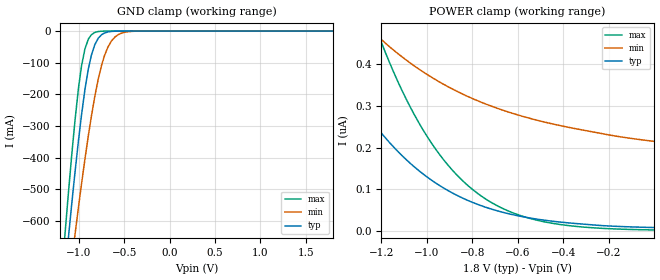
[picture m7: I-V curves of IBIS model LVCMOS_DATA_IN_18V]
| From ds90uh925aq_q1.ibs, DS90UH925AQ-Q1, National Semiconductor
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[Model] LVCMOS_DATA_IN_18V
Model_type Input
Vinh = 1.17V
Vinl = 0.63V
C_comp   6.98pF   6.05pF   8.06pF
[Voltage Range]   1.8V   1.62V   1.98V
[Temperature Range]   25.0   130.0   -40.0
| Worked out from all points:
|   GND clamp passes 1 mA (typ) near -0.64 V on its own axis
[GND Clamp]
-1.8V     -2.96A     -2.635A    -3.228A
-1.147V   -756.9mA   -899mA     -630.1mA
-1.114V   -658.8mA   -819.7mA   -517.7mA
-1.076V   -548.3mA   -728.9mA   -393.4mA
-1.039V   -442.8mA   -640.4mA   -278.7mA
-968.4mV  -265.6mA   -483.8mA   -110.5mA
-892.8mV  -119mA     -330.2mA   -25.29mA
-822.6mV  -43.26mA   -207.4mA   -4.329mA
-747mV    -11.35mA   -107.3mA   -370.4uA
-676.8mV  -2.58mA    -49.95mA   -28.17uA
-493.2mV  -19.24uA   -3.72mA    -1.533uA
1.796V    8.087nA    0A         1.419nA
[POWER Clamp]
-1.8V     917.5nA    912.1nA    12.77uA
-1.487V   487.3nA    635.3nA    977.6nA
-1.341V   342.9nA    537.2nA    680.4nA
-1.255V   273.4nA    487.9nA    534.3nA
-1.217V   246.5nA    468.2nA    477.4nA
-1.109V   180.9nA    418.3nA    337.2nA
-1.001V   130.4nA    376.7nA    229nA
-887.4mV  91.16nA    341nA      146nA
-763.2mV  61.12nA    309.9nA    84.9nA
-633.6mV  40.5nA     284.4nA    46.13nA
-487.8mV  26.18nA    262.3nA    22.42nA
-1.8mV    8.156nA    215.3nA    2.396nA
